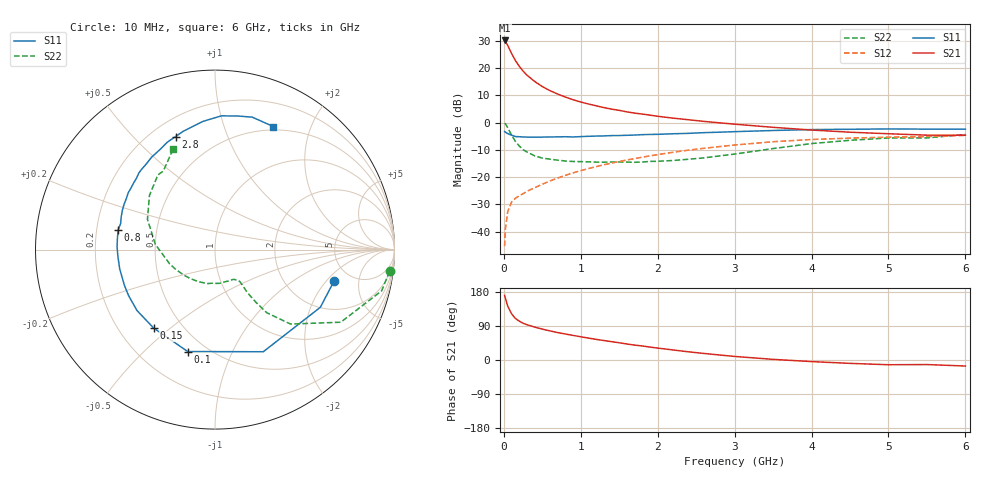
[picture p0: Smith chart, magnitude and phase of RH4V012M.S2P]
! SIEMENS Small Signal Semiconductors
! BFR106
! Si NPN RF Bipolar Junction Transistor in SOT23
! VCE = 4 V  IC = 12 mA
! Common Emitter S-Parameters:  August  1996
# GHz  S  MA  R  50
!  f  S11  S21  S12  S22
! GHz  MAG  ANG  MAG  ANG  MAG  ANG  MAG  ANG
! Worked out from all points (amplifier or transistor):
!   36 points, 10 MHz to 6 GHz, reference 50 ohm
!   highest |S21| = 30.2 dB at 10 MHz (marker M1)
!   |S21| within 3 dB of that: start of sweep to 70.48 MHz
!   unconditionally stable (mu >= 1): 451.4 MHz to 2.092 GHz; 5.3 GHz to end of sweep
!   at 250 MHz: K = 0.77, MSG = 22.5 dB, |S12| = -26.1 dB
!   at 1.4 GHz: K = 1.08, MAG = 8.2 dB, |S12| = -14.9 dB
!   at 6 GHz: K = 1.01, MAG = -0.5 dB, |S12| = -4.7 dB
!   S11 on the Smith chart (normalised r, x): 10 MHz: 3.69, -2.43; 100 MHz: 0.40, -0.69; 150 MHz: 0.35, -0.44; 800 MHz: 0.29, +0.09; 2.8 GHz: 0.29, +0.67; 6 GHz: 0.46, +1.48
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0.01  0.6863 -14.7  32.23 170.7  0.0054 84.1  0.98 -7.1
0.02  0.6692 -28.7  31.18 163.2  0.0111 74.8  0.9564 -13.9
0.05  0.6295 -64.7  26.21 142.4  0.0231 63.7  0.8092 -30.0
0.1  0.5879 -105.0  18.68 122.0  0.0348 51.9  0.5908 -44.6
0.15  0.5549 -128.0  13.79 109.6  0.0409 47.9  0.4538 -50.7
0.2  0.5515 -142.0  10.86 102.6  0.0453 48.9  0.3741 -52.1
0.25  0.5455 -152.0  8.841 97.0  0.0496 50.0  0.3196 -52.8
0.3  0.5426 -158.6  7.455 93.1  0.0548 51.9  0.2889 -52.9
0.4  0.5417 -168.6  5.7 86.9  0.0639 55.4  0.246 -52.4
0.5  0.5423 -175.9  4.59 81.5  0.074 58.0  0.2234 -52.2
0.6  0.546 178.3  3.862 76.8  0.0851 60.1  0.2133 -53.2
0.8  0.5511 168.6  2.943 68.6  0.1077 62.1  0.1973 -57.3
0.9  0.5454 164.6  2.633 64.9  0.1196 62.5  0.1936 -59.5
1.1  0.5612 156.7  2.197 57.8  0.1434 62.7  0.1907 -66.7
1.3  0.5702 150.0  1.889 51.4  0.1685 62.0  0.1878 -74.0
1.6  0.5856 140.9  1.575 42.2  0.2062 59.9  0.1887 -87.6
2.2  0.6248 124.3  1.209 26.5  0.2857 53.5  0.2018 -118.6
2.8  0.6672 109.2  0.993 13.3  0.3629 45.0  0.2446 -153.0
3.5  0.717 95.5  0.82 1.7  0.4461 33.8  0.3341 174.9
4.5  0.7546 80.6  0.667 -8.9  0.5195 17.1  0.4738 140.4
5.5  0.7592 68.5  0.589 -12.0  0.5529 6.0  0.5241 123.3
6  0.7592 64.6  0.587 -15.9  0.5837 -1.7  0.6076 112.5
